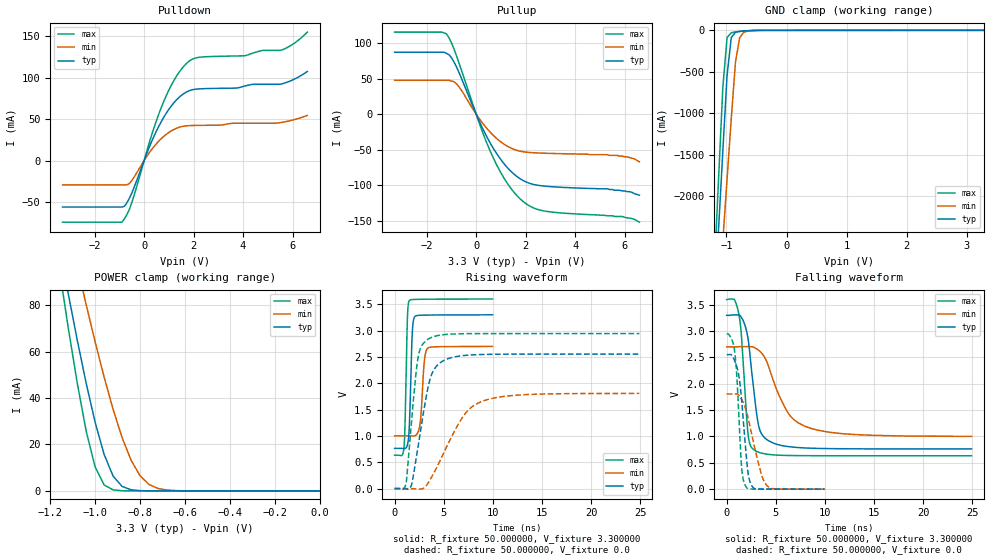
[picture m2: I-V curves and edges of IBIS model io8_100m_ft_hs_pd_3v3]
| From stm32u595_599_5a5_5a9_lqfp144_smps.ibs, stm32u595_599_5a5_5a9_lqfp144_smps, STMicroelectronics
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|   Model io8_100m_ft_hs_pd_3v3
[Model]  io8_100m_ft_hs_pd_3v3
Model_type I/O
Polarity   Non-Inverting
Enable   Active-Low
Vinl =   0.990000V
Vinh =   2.310000V
Vmeas =  1.650000V
Cref =   50.000000pF
Rref =   100.000000M
Vref =   0.0V
C_comp   3.313100pF   3.281800pF   3.354500pF
[Temperature Range]   25.000000   0.140000k   -40.000000
[Pullup Reference]   3.300000V   2.700000V   3.600000V
[Pulldown Reference]   0.0V   0.0V   0.0V
[POWER Clamp Reference]   3.300000V   2.700000V   3.600000V
[GND Clamp Reference]   0.0V   0.0V   0.0V
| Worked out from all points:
|   slope of the pulldown table from 0 to 0.495 V, typ, clamps not added: 14 ohm
|   slope of the pullup table from 0 to 0.495 V, typ, clamps not added: 13.7 ohm
|   GND clamp passes 1 mA (typ) near -0.50 V on its own axis
|   POWER clamp passes 1 mA (typ) near -0.85 V on its own axis
|   rising waveform, R_fixture 50.000000, V_fixture 3.300000: 20-80 % time 245ps typ, 342ps min, 208ps max; typ from 0.764 V to 3.3 V
|   rising waveform, R_fixture 50.000000, V_fixture 0.0: 20-80 % time 1.41ns typ, 3.1ns min, 872ps max; typ from 0 V to 2.55 V
|   falling waveform, R_fixture 50.000000, V_fixture 3.300000: 20-80 % time 959ps typ, 2.51ns min, 626ps max; typ from 3.3 V to 0.764 V
|   falling waveform, R_fixture 50.000000, V_fixture 0.0: 20-80 % time 726ps typ, 1.36ns min, 504ps max; typ from 2.55 V to 0 V
[Pulldown]
|Voltage   I(typ)   I(min)   I(max)
-3.3V     -56.06mA   -29.42mA   -74.35mA
-900mV    -56.06mA   -29.42mA   -74.35mA
-700mV    -51.09mA   -29.42mA   -65.48mA
-500mV    -39.32mA   -24.2mA    -50.88mA
300mV     22.62mA    13.13mA    30.42mA
800mV     52.54mA    29.36mA    71.75mA
1.3V      72.91mA    38.82mA    101.4mA
1.8V      84.02mA    42.13mA    119.4mA
2.2V      86.43mA    42.46mA    124.5mA
5.5V      91.98mA    45.75mA    132.9mA
6.1V      98.6mA     49.6mA     142.1mA
6.6V      107.5mA    54.5mA     155mA
[Pullup]
|Voltage   I(typ)   I(min)   I(max)
-3.3V     87.21mA    47.72mA    115.6mA
-1.2V     85.53mA    47.72mA    112.9mA
-1V       79.42mA    46.66mA    100.4mA
-700mV    59.08mA    38.76mA    72.42mA
100mV     -8.009mA   -5.102mA   -10.2mA
600mV     -42.64mA   -26.6mA    -54.61mA
1.2V      -72.81mA   -43.84mA   -94.18mA
1.9V      -93.37mA   -52.9mA    -122.9mA
2.3V      -98.71mA   -54.23mA   -131.7mA
2.8V      -101.3mA   -54.97mA   -136.5mA
5.7V      -107mA     -58mA      -144mA
6.6V      -114mA     -67mA      -152mA
[GND_clamp]
|Voltage   I(typ)   I(min)   I(max)
-3.3V     -9.848A    -9.957A    -9.458A
-1.2V     -3.312A    -4.013A    -2.863A
-1.13V    -2.381A    -3.274A    -1.769A
-1.06V    -1.452A    -2.535A    -684.8mA
-990mV    -542.9mA   -1.798A    -88.04mA
-920mV    -87.13mA   -1.064A    -28.45mA
-850mV    -22.11mA   -382.4mA   -19.62mA
-780mV    -11.98mA   -86.98mA   -13.73mA
-710mV    -7.63mA    -22.27mA   -8.759mA
-640mV    -4.504mA   -7.781mA   -4.831mA
-360mV    -39.8uA    -178.9uA   -19.56uA
3.28V     83.52uA    56.87uA    102.4uA
[POWER_clamp]
|Voltage   I(typ)   I(min)   I(max)
-3.28V    1.355A     1.167A     1.664A
-1.16V    105.7mA    131.6mA    95.69mA
-1.12V    84.97mA    114mA      70.27mA
-1.08V    65.05mA    96.83mA    46.54mA
-1.04V    46.34mA    80.15mA    25.76mA
-1V       29.51mA    64.13mA    10.3mA
-960mV    15.69mA    48.99mA    2.571mA
-920mV    6.373mA    35.1mA     455.6uA
-840mV    490.7uA    13.24mA    11.36uA
-760mV    27.33uA    2.767mA    276.6nA
-640mV    346.6nA    134.1uA    15.62nA
0V        0A         19.91nA    0A
[Ramp]
| variable   typ   min   max
dV/dt_r  1.53198/1.41046n   1.08378/3.09866n   1.76610/0.87034n
dV/dt_f  1.52118/0.95568n   1.01790/2.50769n   1.77922/0.62411n
R_load = 50.000000
[Rising Waveform]
R_fixture= 50.000000
V_fixture= 3.300000
V_fixture_min= 2.700000
V_fixture_max= 3.600000
|time   V(typ)   V(min)   V(max)
0s        763.9mV    1.001V     633.7mV
961ps     759.7mV    1.001V     793.7mV
1.301ns   826.6mV    1.001V     3.215V
1.481ns   1.121V     1.001V     3.564V
1.782ns   2.883V     998.9mV    3.589V
2.042ns   3.263V     1.001V     3.592V
2.563ns   3.291V     1.197V     3.594V
3.043ns   3.294V     2.443V     3.595V
3.363ns   3.295V     2.663V     3.596V
9.97ns    3.299V     2.699V     3.599V
[Rising Waveform]
R_fixture= 50.000000
V_fixture= 0.0
V_fixture_min= 0.0
V_fixture_max= 0.0
|time   V(typ)   V(min)   V(max)
0s        6.698uV    6.792uV    3.581uV
1.151ns   -8.748mV   18.83uV    86.42mV
1.702ns   59.79mV    -894.4nV   1.225V
2.452ns   870.7mV    -9.575mV   2.55V
3.453ns   1.964V     118.8mV    2.842V
3.954ns   2.242V     282.3mV    2.884V
5.005ns   2.432V     679.3mV    2.923V
7.057ns   2.526V     1.392V     2.94V
8.809ns   2.545V     1.649V     2.943V
24.92ns   2.553V     1.806V     2.943V
[Falling Waveform]
R_fixture= 50.000000
V_fixture= 3.300000
V_fixture_min= 2.700000
V_fixture_max= 3.600000
|time   V(typ)   V(min)   V(max)
0s        3.299V     2.699V     3.599V
1.251ns   3.305V     2.704V     3.307V
1.502ns   3.259V     2.705V     2.916V
2.202ns   2.821V     2.705V     1.003V
2.853ns   1.729V     2.684V     737.7mV
3.253ns   1.203V     2.637V     701.8mV
3.804ns   988.1mV    2.52V      674mV
6.106ns   812.7mV    1.49V      640.1mV
7.908ns   783.1mV    1.198V     635.7mV
24.92ns   763.9mV    1.001V     633.7mV
[Falling Waveform]
R_fixture= 50.000000
V_fixture= 0.0
V_fixture_min= 0.0
V_fixture_max= 0.0
|time   V(typ)   V(min)   V(max)
0s        2.553V     1.806V     2.943V
800.8ps   2.443V     1.806V     2.629V
1.041ns   2.314V     1.81V      2.113V
1.522ns   1.685V     1.706V     406.1mV
1.962ns   697.3mV    1.503V     45.83mV
2.222ns   256.4mV    1.315V     7.219mV
2.523ns   75.06mV    1.063V     2.679mV
3.483ns   2.244mV    314.5mV    1.144mV
4.124ns   1.353mV    63.69mV    873.9uV
9.97ns    6.698uV    6.792uV    3.581uV
